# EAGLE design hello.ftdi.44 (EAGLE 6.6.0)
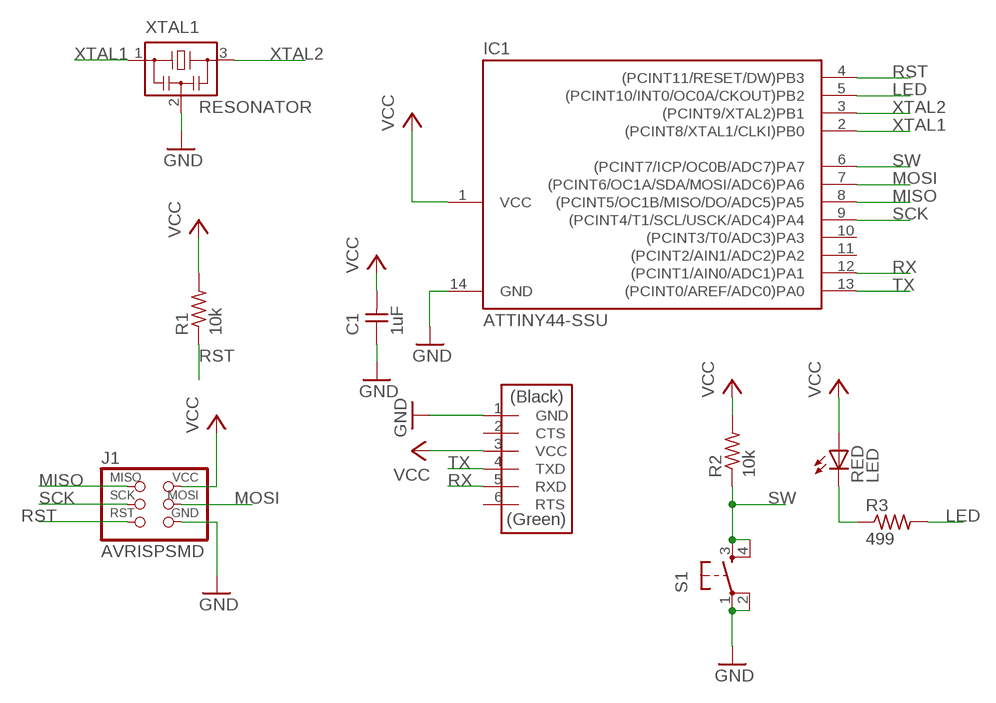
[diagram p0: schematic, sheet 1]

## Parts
C1  1uF  CAP-UNPOLARIZEDFAB  [C1206FAB]
IC1  ATTINY44-SSU  [SOIC14]
J1  AVRISPSMD  [2X03SMD]
J2  FTDI-SMD-HEADER  [1X06SMD]
R1  10k  RES-US1206FAB  [R1206FAB]
R2  10k  RES-US1206FAB  [R1206FAB]
R3  499  RES-US1206FAB  [R1206FAB]
RED  LED  [LED1206]
S1  6MM_SWITCH6MM_SWITCH  [6MM_SWITCH]
XTAL1  RESONATOR  [EFOBM]

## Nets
GND: C1.1 IC1.14(GND) J1.6(GND) J2.1(GND) S1.1(P) S1.2(P1) XTAL1.2
LED: IC1.5((PCINT10/INT0/OC0A/CKOUT)PB2) R3.2
MISO: IC1.8((PCINT5/OC1B/MISO/DO/ADC5)PA5) J1.1(MISO)
MOSI: IC1.7((PCINT6/OC1A/SDA/MOSI/ADC6)PA6) J1.4(MOSI)
N$1: R3.1 RED.2(C)
RST: IC1.4((PCINT11/RESET/DW)PB3) J1.5(RST) R1.1
RX: IC1.12((PCINT1/AIN0/ADC1)PA1) J2.5(RXD)
SCK: IC1.9((PCINT4/T1/SCL/USCK/ADC4)PA4) J1.3(SCK)
SW: IC1.6((PCINT7/ICP/OC0B/ADC7)PA7) R2.1 S1.3(S) S1.4(S1)
TX: IC1.13((PCINT0/AREF/ADC0)PA0) J2.4(TXD)
VCC: C1.2 IC1.1(VCC) J1.2(VCC) J2.3(VCC) R1.2 R2.2 RED.1(A)
XTAL1: IC1.2((PCINT8/XTAL1/CLKI)PB0) XTAL1.1
XTAL2: IC1.3((PCINT9/XTAL2)PB1) XTAL1.3
Unconnected: IC1.10((PCINT3/T0/ADC3)PA3) IC1.11((PCINT2/AIN1/ADC2)PA2) J2.2(CTS) J2.6(RTS)

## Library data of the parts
C1 = fab:CAP-UNPOLARIZED
IC1 = fab:ATTINY44
J1 = fab:AVRISP
J2 = fab:FTDI-SMD-HEADER
R1-R3 = fab:RES-US: Resistor (US Symbol)
RED = fab:LED: LED
S1 = fab:6MM_SWITCH: OMRON SWITCH
XTAL1 = fab:RESONATOR

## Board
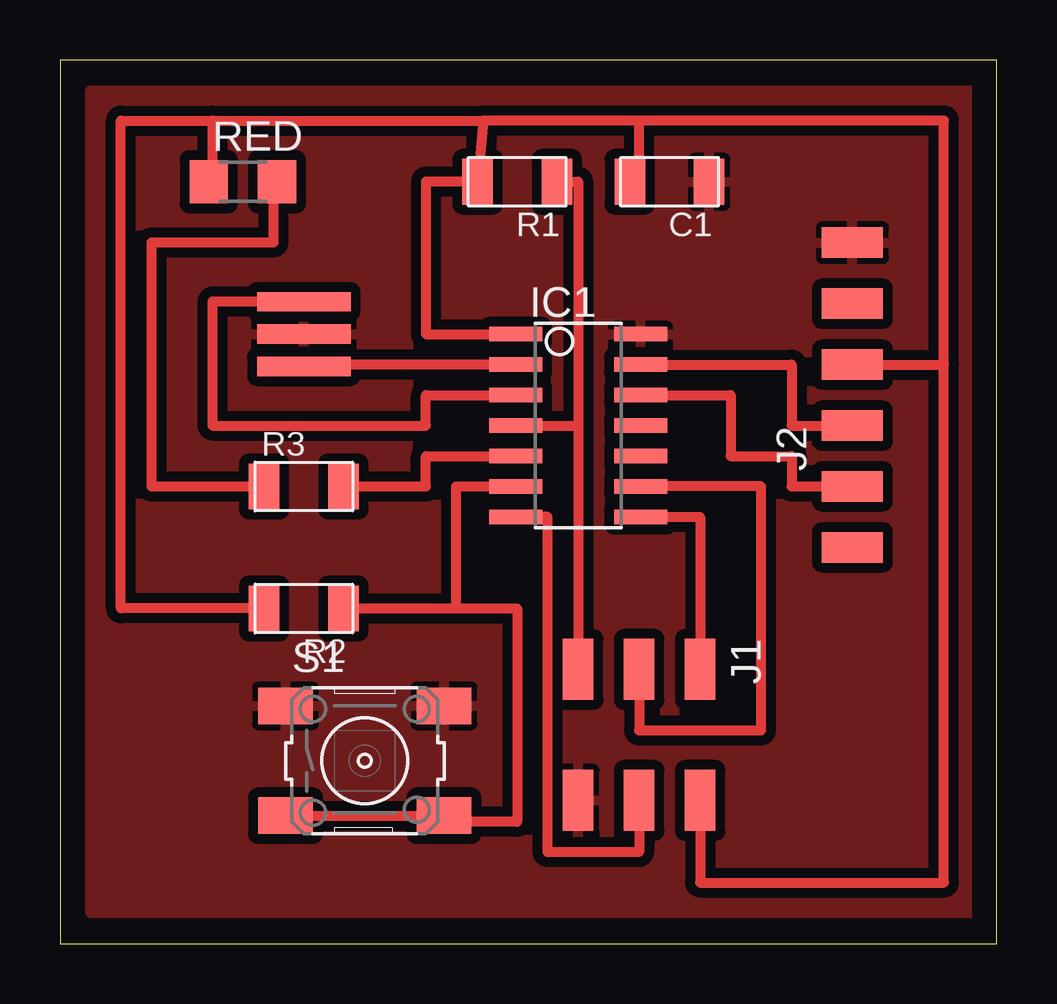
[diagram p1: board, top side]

Size 39.04 x 36.82 mm. Coordinates in mm from the lower left corner, seen from the top.
Outline: 0,0 39.04,0 39.04,36.82 0,36.82 0,0
Copper layers (1*16): Top 0.035mm / dielectric 1.5mm / Bottom 0.035mm
Design rules "fabmodule": minimum track width 10mil, minimum drill 0.4mm, track to track 0.42mm, track to pad 0.42mm, pad to pad 0.42mm, via to via 0.42mm, smd to smd 0.42mm, copper to edge 40mil, drill to drill 0.8mm, minimum pad ring 10mil, minimum via ring 8mil, stop-mask expansion 4mil, vias tented up to drill 0mil, thermal gap 10mil

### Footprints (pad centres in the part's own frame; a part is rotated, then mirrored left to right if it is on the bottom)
C1206FAB = smd 1.27 x 1.905: 1 -1.651,0; 2 1.651,0
SOIC14 = smd 0.61 x 2.21: 1 -3.81,-2.603; 2 -2.54,-2.603; 3 -1.27,-2.603; 4 0,-2.603; 5 1.27,-2.603; 6 2.54,-2.603; 7 3.81,-2.603; 8 3.81,2.603; 9 2.54,2.603; 10 1.27,2.603; 11 0,2.603; 12 -1.27,2.603; 13 -2.54,2.603; 14 -3.81,2.603
2X03SMD = smd 2.54 x 1.27: 1 -2.54,2.54; 2 2.92,2.54; 3 -2.54,0; 4 2.92,0; 5 -2.54,-2.54; 6 2.92,-2.54
1X06SMD = smd 2.54 x 1.27: 1 0,6.35; 2 0,3.81; 3 0,1.27; 4 0,-1.27; 5 0,-3.81; 6 0,-6.35
R1206FAB = smd 1.27 x 1.905: 1 -1.651,0; 2 1.651,0
LED1206 = smd 1.6 x 1.803: 1 -1.422,0; 2 1.422,0
6MM_SWITCH = smd 2.286 x 1.524: 1 -3.302,2.286; 2 3.302,2.286; 3 -3.302,-2.286; 4 3.302,-2.286
EFOBM = smd 0.8 x 3.9: 1 -1.35,0; 2 0,0; 3 1.35,0

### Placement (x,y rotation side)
C1  25.4,31.75 180 top
IC1  21.59,21.59 270 top
J1  24.13,8.89 270 top
J2  33.02,22.86 0 top
R1  19.05,31.75 180 top
R2  10.16,13.97 180 top
R3  10.16,19.05 0 top
RED  7.62,31.75 0 top
S1  12.7,7.62 0 top
XTAL1  10.16,25.4 90 top

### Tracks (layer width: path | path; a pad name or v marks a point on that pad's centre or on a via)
GND
  Top 0.406: S1.2 16.51,9.91 16.51,10.16
  pour Top: 1.27,35.56 38.1,35.56 38.1,1.27 1.27,1.27
LED
  Top 0.254: 11.43,19.05 R3.2
  Top 0.406: R3.2 15.24,19.05 15.24,20.32 IC1.5
MISO
  Top 0.406: IC1.8 26.67,17.78 J1.1
MOSI
  Top 0.406: J1.4 24.13,3.81 20.32,3.81 20.32,17.78 IC1.7
N$1
  Top 0.406: RED.2 8.89,31.75 8.89,29.21 3.81,29.21 3.81,19.05 R3.1 8.89,19.05
RST
  Top 0.406: R1.1 21.59,31.75 21.59,21.59 | 21.59,21.59 J1.5 | IC1.4 21.59,21.59
RX
  Top 0.406: IC1.12 27.94,22.86 27.94,20.32 30.48,20.32 30.48,19.05 J2.5
SCK
  Top 0.406: J1.3 24.13,8.89 29.21,8.89 29.21,19.05 IC1.9
SW
  Top 0.406: S1.3 S1.4 16,5.08 19.05,5.08 19.05,13.97 16.51,13.97 | R2.1 16.51,13.97 | 16.51,13.97 16.51,19.05 IC1.6
TX
  Top 0.406: IC1.13 30.48,24.13 30.48,21.59 J2.4
VCC
  Top 0.406: RED.1 6.35,31.75 6.35,34.29 | 6.35,34.29 17.63,34.29 | 17.63,34.29 R1.2 15.24,31.75 15.24,25.4 IC1.1 19.05,25.4 | C1.2 24.13,31.75 24.13,34.29 | 24.13,34.29 17.63,34.29 | J2.3 36.83,24.13 | 36.83,24.13 36.83,34.29 24.13,34.29 | R2.2 2.54,13.97 2.54,34.29 6.35,34.29 | J1.2 26.67,2.54 36.83,2.54 36.83,24.13
XTAL1
  Top 0.406: IC1.2 10.16,24.13 XTAL1.1
XTAL2
  Top 0.406: XTAL1.3 6.35,26.75 6.35,21.59 15.24,21.59 15.24,22.86 IC1.3 19.05,22.86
